FUNCTION_BLOCK FB_CylinderTempRecord EXTENDS FB_CylinderTemp
VAR_INPUT
	bRecordStart		: BOOL;
	tiIntervalTime		: TIME;
END_VAR
VAR_OUTPUT
	bRecordDone			: BOOL;
	lrTemps				: ARRAY[1..100] OF LREAL;
END_VAR
VAR
	IntervalTimer		: TON;
	iIndex				: INT;
END_VAR

// =========================================================
;
// =========================================================

METHOD PUBLIC M_Record
VAR_INPUT
END_VAR
// =========================================================
	// Recording array filled
	
bRecordDone := (iIndex = 100);

// =========================================================
	// Recording temperatures
	
IF bRecordStart AND NOT bRecordDone AND NOT IntervalTimer.Q THEN
	IntervalTimer( IN := TRUE, PT := tiIntervalTime );
END_IF

IF IntervalTimer.Q THEN
	IntervalTimer( IN := FALSE );
	iIndex := iIndex + 1;
	lrTemps[iIndex] := lrTempCurrent;
END_IF

// =========================================================
END_METHOD

METHOD PUBLIC M_Reset
VAR_INPUT
END_VAR
// =========================================================
	// Reset
	
SUPER^.M_Reset();					// Calling method M_Reset of base class FB_Cylinder via 'SUPER^.'

FOR iIndex := 1 TO 100 BY 1 DO
	lrTemps[iIndex] := 0;
END_FOR

iIndex := 0;

// =========================================================
END_METHOD

END_FUNCTION_BLOCK
